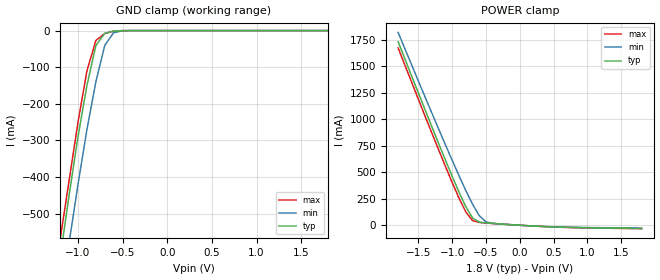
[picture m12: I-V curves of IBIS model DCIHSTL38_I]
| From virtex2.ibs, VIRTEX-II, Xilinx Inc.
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|   Model DCIHSTL38_I
[Model]   DCIHSTL38_I
Model_type   Input
Vinh = 1.2V
Vinl = 1.0V
Polarity   Non-Inverting
C_comp   7.00pF   6.00pF   8.00pF
[Temperature Range]   25.00   100.00   0.000
[Voltage Range]   1.80V   1.70V   1.90V
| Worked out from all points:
|   GND clamp passes 1 mA (typ) near -0.57 V on its own axis
|   POWER clamp passes 1 mA (typ) near -0.02 V on its own axis
[GND_clamp]
| voltage   I(typ)   I(min)   I(max)
-1.8V     -1.65A     -1.74A     -1.6A
-1.2V     -620mA     -740mA     -570mA
-1.1V     -450mA     -580mA     -410mA
-1V       -290mA     -420mA     -250mA
-900mV    -150mA     -270mA     -110mA
-800mV    -40.97mA   -140mA     -27.17mA
-700mV    -7.54mA    -40.17mA   -8.08mA
-600mV    -1.39mA    -5.57mA    -1.57mA
-500mV    -120uA     -660uA     -120uA
1.8V      34.27pA    98.88nA    22.46pA
[POWER_clamp]
| voltage   I(typ)   I(min)   I(max)
-1.8V     1.732A     1.82A      1.673A
-1.4V     1.087A     1.208A     1.027A
-1V       460.5mA    611.5mA    401.8mA
-900mV    312.7mA    467.7mA    256.1mA
-800mV    176mA      328.8mA    126.3mA
-700mV    69.28mA    199.2mA    44.33mA
-600mV    29.76mA    90.8mA     26.43mA
-500mV    22.34mA    31.4mA     20.7mA
-400mV    17.48mA    17.72mA    16.35mA
500mV     -15.81mA   -14.66mA   -16.03mA
1.8V      -29.89mA   -27.07mA   -32.03mA
